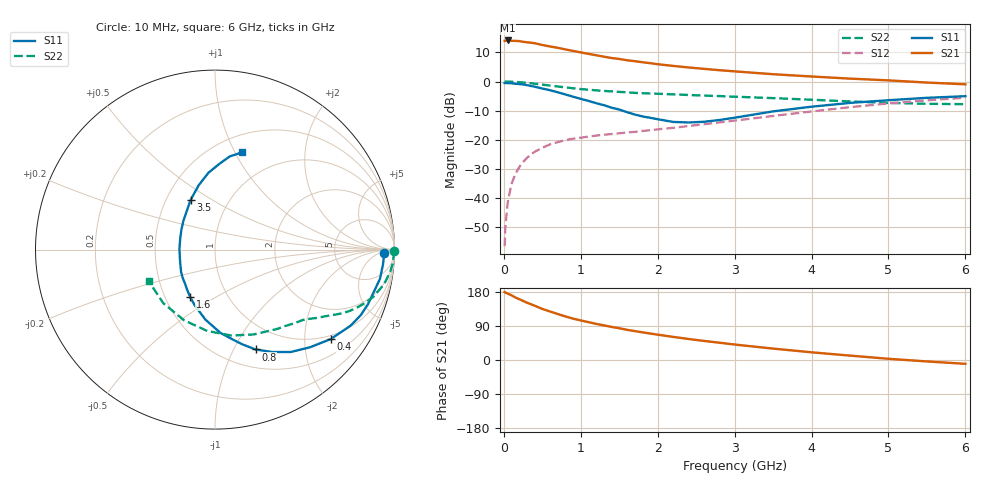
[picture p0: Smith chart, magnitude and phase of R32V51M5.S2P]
! SIEMENS Small Signal Semiconductors
! BFR181
! Si NPN RF Bipolar Junction Transistor in SOT23
! VCE = 2.5 V  IC = 1.5 mA
! Common Emitter S-Parameters:  May  1996
# GHz  S  MA  R  50
!  f  S11  S21  S12  S22
! GHz  MAG  ANG  MAG  ANG  MAG  ANG  MAG  ANG
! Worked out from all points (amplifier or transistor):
!   36 points, 10 MHz to 6 GHz, reference 50 ohm
!   highest |S21| = 14.1 dB at 50 MHz (marker M1)
!   |S21| within 3 dB of that: start of sweep to 786.9 MHz
!   unconditionally stable (mu >= 1): 1.733 GHz to 3.497 GHz
!   at 250 MHz: K = 0.20, MSG = 20.6 dB, |S12| = -27.6 dB
!   at 1.4 GHz: K = 0.88, MSG = 13.0 dB, |S12| = -18.0 dB
!   at 6 GHz: K = 0.86, MSG = 2.3 dB, |S12| = -5.6 dB
!   S11 on the Smith chart (normalised r, x): 10 MHz: 31, -9; 400 MHz: 0.90, -2.66; 800 MHz: 0.70, -1.22; 1.6 GHz: 0.67, -0.39; 3.5 GHz: 0.66, +0.40; 6 GHz: 0.67, +1.06
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0.01  0.9433 -1.0  4.981 179.2  0.0015 81.1  0.9984 -0.5
0.02  0.9425 -1.9  4.985 178.0  0.0032 84.2  0.9974 -1.0
0.05  0.9396 -5.0  5.065 175.2  0.0084 87.8  0.9952 -2.3
0.1  0.9337 -10.0  4.989 170.7  0.0176 84.9  0.9928 -4.6
0.15  0.9164 -14.7  4.978 165.0  0.0259 80.1  0.9849 -6.9
0.2  0.9051 -19.6  4.94 160.6  0.0339 77.9  0.9738 -9.1
0.3  0.8667 -29.2  4.721 151.3  0.0491 72.7  0.9491 -13.0
0.4  0.8152 -37.7  4.548 143.3  0.0623 67.7  0.9197 -16.7
0.5  0.7591 -45.8  4.236 134.8  0.0732 63.5  0.8844 -19.8
0.6  0.7096 -53.5  3.993 128.0  0.0834 59.9  0.8527 -22.4
0.8  0.6006 -67.9  3.556 115.0  0.099 54.5  0.7937 -26.5
0.9  0.5486 -74.0  3.353 109.1  0.1046 52.7  0.7663 -28.1
1.1  0.4648 -86.3  2.986 99.9  0.1137 50.7  0.7231 -30.8
1.3  0.3937 -97.8  2.671 91.4  0.1222 49.3  0.6904 -33.1
1.6  0.2987 -117.6  2.317 79.7  0.1337 49.1  0.6536 -36.2
1.9  0.2391 -139.0  2.067 69.9  0.146 50.6  0.6229 -39.3
2.2  0.2029 -164.2  1.854 61.0  0.1606 51.7  0.6022 -43.0
2.8  0.2185 148.8  1.566 45.7  0.199 53.5  0.5633 -51.5
3.5  0.3076 116.3  1.335 30.1  0.2568 52.5  0.5195 -65.5
4.5  0.4302 94.8  1.122 11.6  0.3633 45.6  0.4554 -95.4
5.5  0.5255 81.0  0.96 -3.8  0.4763 33.1  0.4149 -134.0
6  0.561 74.7  0.896 -10.1  0.527 25.5  0.4089 -154.5
